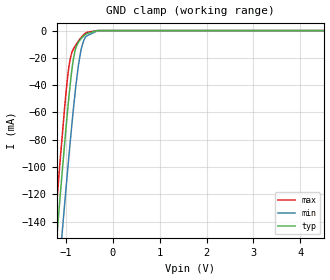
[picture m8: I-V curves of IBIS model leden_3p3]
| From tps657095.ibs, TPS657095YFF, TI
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|   leden_3p3 Model
[Model]   leden_3p3
Model_type   Input
Vinl = 0.4
Vinh = 1.2
|   typ   min   max
|   (nom PVT)   (fast PVT)   (slow PVT)
C_comp   1.765e-12   1.702e-12   1.852e-12
| Where nom  PVT is Nominal Process, 3.3V, 27C
|   Fast PVT is Strong Process,  3.6V, -40C
|   Slow PVT is Weak Process,   3V, 125C
[Voltage Range]   3.3   3   3.6
|Junction Temperature
[Temperature Range]   27   125   -40
[Power Clamp Reference]   3.3   3   3.6
[GND Clamp Reference]   0   0   0
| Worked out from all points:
|   GND clamp passes 1 mA (typ) near -0.43 V on its own axis
[GND Clamp]
|   Voltage   I(typ)   I(min)   I(max)
-3.3V     -1.127A    -1.134A    -1.132A
-1.297V   -195.8mA   -237.8mA   -171.6mA
-1.14V    -128.7mA   -172.6mA   -102.5mA
-1.119V   -120mA     -164.1mA   -93.63mA
-1.025V   -81.87mA   -126.3mA   -55.51mA
-957mV    -56.21mA   -100mA     -32.18mA
-898.8mV  -36.49mA   -78.3mA    -19.23mA
-828.3mV  -18.57mA   -53.58mA   -12.77mA
-678mV    -6.052mA   -14.16mA   -5.253mA
-564mV    -2.347mA   -4.068mA   -1.417mA
-246mV    -1.291uA   -26.63uA   -39.76nA
6.6V      0A         0A         0A
[POWER Clamp]
|   Voltage   I(typ)   I(min)   I(max)
-3.3V     0A         0A         0A
0V        0A         0A         0A
6.6V      0A         0A         0A
